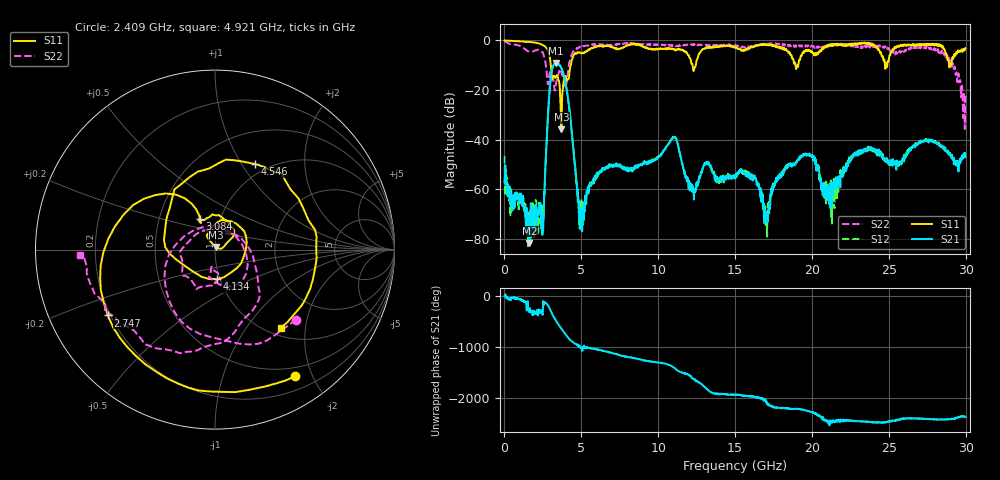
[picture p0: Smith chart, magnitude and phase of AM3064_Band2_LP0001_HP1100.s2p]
# Hz S DB R 50.0
!freq dBS11 angS11 dBS21 angS21 dBS12 angS12 dBS22 angS22
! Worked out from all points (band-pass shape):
!   1600 points, 10 MHz to 29.98 GHz, reference 50 ohm
!   highest |S21| = -9.07 dB at 3.328 GHz (marker M1); lowest = -81.7 dB at 1.622 GHz (marker M2)
!   |S21| within 3 dB of the highest: 3.079 GHz to 3.762 GHz (683.2 MHz wide, 20 % of centre)
!   lowest |S11| = -35.9 dB at 3.703 GHz (marker M3), VSWR 1.03, Z = 50.6 + j1.5 ohm
!   |S11| at or under -10 dB: 3.015 GHz to 4.318 GHz (1.302 GHz wide, 35.5 % of centre); 12.24 GHz to 12.44 GHz (204.1 MHz wide, 1.65 % of centre); 18.93 GHz to 19.11 GHz (179.6 MHz wide, 0.944 % of centre)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
!   |S22| runs from -35.7 to -0.2 dB; largest |S21 - S12| = 0.0089
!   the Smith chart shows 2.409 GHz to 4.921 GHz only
!   S11 on the Smith chart (normalised r, x): 2.409 GHz: 0.38, -1.75; 2.747 GHz: 0.19, -0.27; 3.084 GHz: 0.80, +0.28; 4.134 GHz: 0.97, -0.33; 4.546 GHz: 0.87, +1.15; 4.921 GHz: 1.14, -1.47
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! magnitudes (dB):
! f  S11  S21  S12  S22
! 10 MHz  0.0  -57.2  -46.8  -0.2
! 1.622 GHz  -0.6  -81.7  -71.8  -4.6
! 2.409 GHz  -1.6  -76.0  -73.6  -4.5
! 2.747 GHz  -3.1  -39.9  -39.8  -13.0
! 3.084 GHz  -14.5  -11.9  -11.9  -15.5
! 3.328 GHz  -14.8  -9.1  -9.1  -18.6
! 3.703 GHz  -35.9  -11.1  -11.2  -12.7
! 4.134 GHz  -15.7  -23.6  -23.5  -12.7
! 4.546 GHz  -5.6  -47.8  -47.5  -4.0
! 4.921 GHz  -4.9  -69.8  -69.7  -2.4
! 5.015 GHz  -5.3  -71.3  -63.9  -2.6
! 6.439 GHz  -2.6  -52.0  -51.5  -1.7
! 10 GHz  -3.5  -47.1  -47.1  -1.7
! 12.32 GHz  -12.0  -64.2  -59.6  -1.7
! 15 GHz  -2.7  -54.7  -54.3  -1.9
! 17.03 GHz  -1.7  -71.2  -72.1  -1.3
! 19.99 GHz  -4.5  -46.7  -47.0  -2.1
! 21.32 GHz  -2.2  -59.3  -62.8  -1.8
! 22.91 GHz  -1.2  -45.0  -45.1  -2.7
! 25 GHz  -8.1  -48.6  -48.7  -3.1
! 28.56 GHz  -3.2  -42.9  -42.6  -4.9
! 29.98 GHz  -3.1  -47.1  -46.0  -21.7
